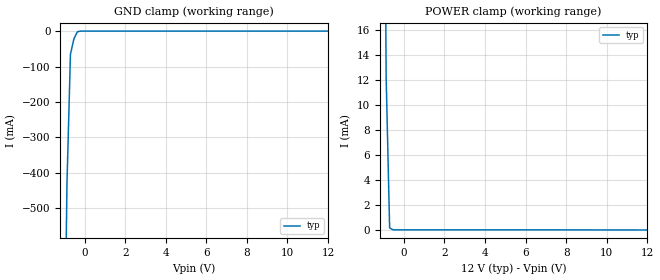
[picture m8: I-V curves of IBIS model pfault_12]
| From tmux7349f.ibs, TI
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| pfault_12
[Model]   pfault_12
Model_type   Input
Vinl = 0.8
Vinh = 1.3
|   typ   min   max
C_comp   1.598234e-11   NA   NA
[Voltage Range]   12   NA   NA
[Temperature Range]   27   NA   NA
[Power Clamp Reference]   12   NA   NA
[GND Clamp Reference]   0   NA   NA
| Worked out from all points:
|   GND clamp passes 1 mA (typ) near -0.29 V on its own axis
|   POWER clamp passes 1 mA (typ) near -0.72 V on its own axis
[GND Clamp]
|   Voltage   I(typ)   I(min)   I(max)
-5V       -27.52A    NA         NA
-1.051V   -1.201A    NA         NA
-878.8mV  -431.3mA   NA         NA
-707.1mV  -65.37mA   NA         NA
-535.4mV  -21.79mA   NA         NA
-363.6mV  -1.787mA   NA         NA
-191.9mV  -5.123uA   NA         NA
12V       9.989uA    NA         NA
[POWER Clamp]
|   Voltage   I(typ)   I(min)   I(max)
-5V       1.413A     NA         NA
-1.05V    55.75mA    NA         NA
-878.8mV  12.23mA    NA         NA
-707.1mV  168.8uA    NA         NA
-535.4mV  10.24uA    NA         NA
12V       -210.6pA   NA         NA
